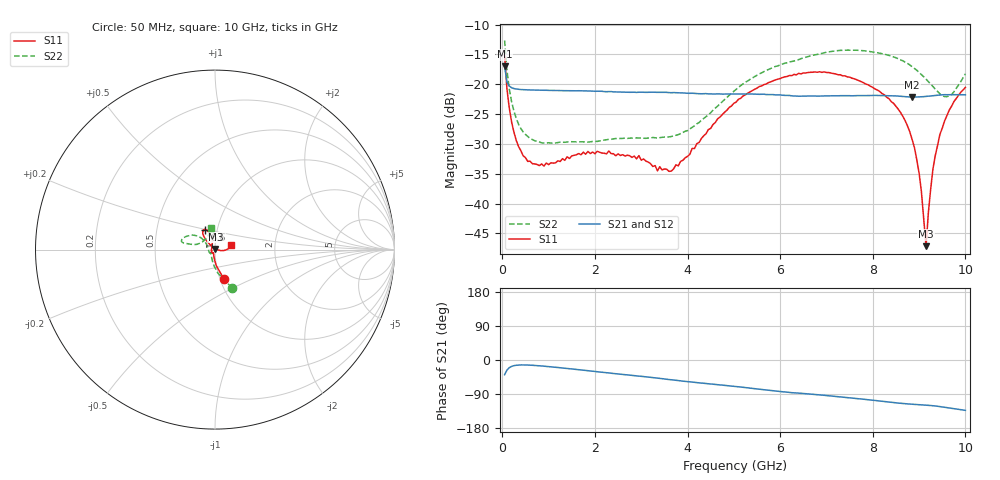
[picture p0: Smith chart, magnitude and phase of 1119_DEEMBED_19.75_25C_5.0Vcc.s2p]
!Hittite Microwave Corp.
!Digital Attenuator/PhaseShifter Rev 1.4.0
!Filename: C:\DATA\DATA\1119_DEEMBED_19.75_25C_5.0Vcc.s2p
!VNA ID: Agilent Technologies,N5224A,MY51441122,A.10.45.03
!Device type:
!2 Port Calibration.
!Temp(C): 25
!Lot Number:
!Serial Number:
!Operator:
!Misc:
!Attenuator:  19.750
# GHZ S DB R 50.0
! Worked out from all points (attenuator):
!   200 points, 50 MHz to 10 GHz, reference 50 ohm
!   highest |S21| = -16.99 dB at 50 MHz (marker M1); lowest = -22.1 dB at 8.85 GHz (marker M2)
!   lowest |S11| = -47.1 dB at 9.15 GHz (marker M3), VSWR 1.01, Z = 50.2 + j0.399 ohm
!   |S11| at or under -10 dB: start of sweep to end of sweep
!   |S22| runs from -29.9 to -12.7 dB; largest |S21 - S12| = 0.00029
!   S11 on the Smith chart (normalised r, x): 50 MHz: 1.05, -0.36; 6.6 GHz: 0.87, +0.20; 10 GHz: 1.20, +0.06
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0.05  -15.21 -72.9  -16.99 -38.8  -16.99 -38.8  -12.65 -66.1
0.1  -20.72 -84.8  -19.58 -26.8  -19.58 -26.8  -17.60 -83.2
0.2  -26.28 -95.0  -20.57 -16.9  -20.58 -16.9  -22.87 -99.8
0.35  -30.41 -103.9  -20.84 -13.3  -20.84 -13.3  -26.67 -113.9
0.55  -32.93 -113.9  -20.94 -13.3  -20.93 -13.3  -28.75 -125.4
0.9  -33.71 -122.6  -21.00 -16.3  -21.00 -16.3  -29.85 -134.5
1.75  -31.38 -134.0  -21.10 -26.9  -21.10 -26.9  -29.65 -139.1
3.4  -33.82 -171.3  -21.35 -48.5  -21.36 -48.6  -28.95 -171.3
3.8  -33.68 146.9  -21.42 -54.3  -21.43 -54.4  -28.44 172.9
5.05  -22.99 107.4  -21.62 -70.1  -21.64 -70.1  -20.85 139.9
6.6  -18.03 116.8  -21.97 -89.4  -21.99 -89.4  -15.36 153.7
6.7  -17.98 117.9  -21.96 -90.5  -21.97 -90.5  -15.14 154.8
7.5  -18.80 126.8  -21.91 -99.9  -21.92 -100.0  -14.28 164.1
8.35  -22.41 132.8  -21.92 -111.0  -21.92 -111.0  -15.16 168.0
8.85  -29.26 134.1  -22.14 -116.6  -22.15 -116.6  -17.05 167.5
8.999999  -34.87 131.2  -22.11 -117.7  -22.12 -117.7  -18.00 167.0
9.15  -47.14 64.8  -22.03 -119.0  -22.04 -119.0  -19.13 165.0
9.2  -41.57 7.7  -21.98 -119.5  -22.00 -119.6  -19.56 163.7
9.3  -34.16 -8.8  -21.90 -120.7  -21.92 -120.8  -20.37 159.7
9.45  -28.38 -9.3  -21.78 -123.1  -21.79 -123.0  -21.61 149.3
9.7  -23.71 -0.1  -21.74 -127.4  -21.75 -127.4  -21.72 121.4
10  -20.53 14.5  -21.77 -132.9  -21.77 -132.9  -18.24 99.8
